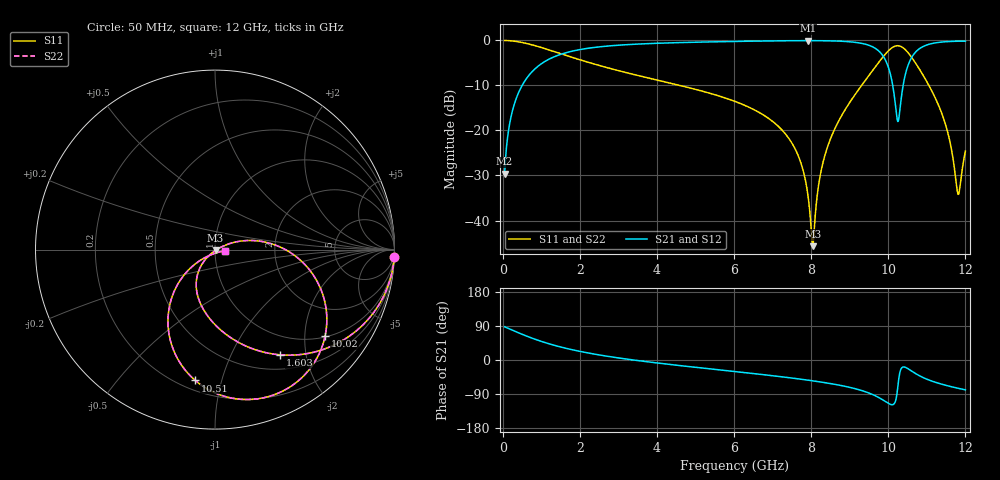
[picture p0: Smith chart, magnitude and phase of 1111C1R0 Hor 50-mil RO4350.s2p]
# GHz S MA R 50
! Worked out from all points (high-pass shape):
!   1601 points, 50 MHz to 12 GHz, reference 50 ohm
!   highest |S21| = -0.05 dB at 7.915 GHz (marker M1); lowest = -29.6 dB at 50 MHz (marker M2)
!   |S21| within 3 dB of the highest: 1.52 GHz to 9.83 GHz (8.31 GHz wide, 146 % of centre); 10.66 GHz to end of sweep
!   lowest |S11| = -45.7 dB at 8.042 GHz (marker M3), VSWR 1.01, Z = 50.3 - j0.428 ohm
!   |S11| at or under -10 dB: 4.595 GHz to 9.308 GHz (4.713 GHz wide, 67.8 % of centre); 11.05 GHz to end of sweep
!   |S22| runs from -45.7 to 0.0 dB; largest |S21 - S12| = 0
!   S11 on the Smith chart (normalised r, x): 50 MHz: 1, -50; 1.603 GHz: 0.70, -1.57; 10.02 GHz: 1.03, -2.53; 10.51 GHz: 0.26, -0.83; 12 GHz: 1.12, -0.01
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0.05  0.9994 -2.3  0.0331 87.7  0.0331 87.7  0.9994 -2.3
0.2217813  0.9894 -10.0  0.1453 80.0  0.1453 80.0  0.9894 -10.0
0.4906563  0.9511 -21.6  0.3086 68.4  0.3086 68.4  0.9511 -21.6
1.6035  0.6904 -58.2  0.7224 31.8  0.7224 31.8  0.6904 -58.2
2.044156  0.6021 -68.0  0.7972 21.9  0.7972 21.9  0.6021 -68.0
4.038312  0.3602 -98.0  0.9309 -8.2  0.9309 -8.2  0.3602 -98.0
6.025  0.2103 -119.8  0.9748 -30.5  0.9748 -30.5  0.2103 -119.8
7.369375  0.08747 -133.5  0.992 -46.0  0.992 -46.0  0.08747 -133.5
7.914594  0.01934 -128.7  0.9946 -53.1  0.9946 -53.1  0.01934 -128.7
8.019156  0.00615 -88.3  0.9945 -54.6  0.9945 -54.6  0.00615 -88.3
8.041562  0.005187 -55.1  0.9944 -54.9  0.9944 -54.9  0.005187 -55.1
8.250687  0.03434 22.0  0.9931 -58.1  0.9931 -58.1  0.03434 22.0
8.5345  0.08766 22.4  0.9884 -62.8  0.9884 -62.8  0.08766 22.4
9.512906  0.4161 -1.9  0.8787 -87.7  0.8787 -87.7  0.4161 -1.9
10.01331  0.7746 -37.3  0.4877 -115.0  0.4877 -115.0  0.7746 -37.3
10.02078  0.7801 -38.1  0.4763 -115.4  0.4763 -115.4  0.7801 -38.1
10.25231  0.8738 -67.1  0.1258 -66.7  0.1258 -66.7  0.8738 -67.1
10.50625  0.7371 -98.6  0.5194 -22.7  0.5194 -22.7  0.7371 -98.6
10.805  0.4818 -123.0  0.8082 -41.4  0.8082 -41.4  0.4818 -123.0
11.38756  0.1546 -143.6  0.9602 -63.9  0.9602 -63.9  0.1546 -143.6
11.80581  0.01977 -81.7  0.9799 -74.5  0.9799 -74.5  0.01977 -81.7
12  0.05882 -6.1  0.9804 -78.8  0.9804 -78.8  0.05882 -6.1
